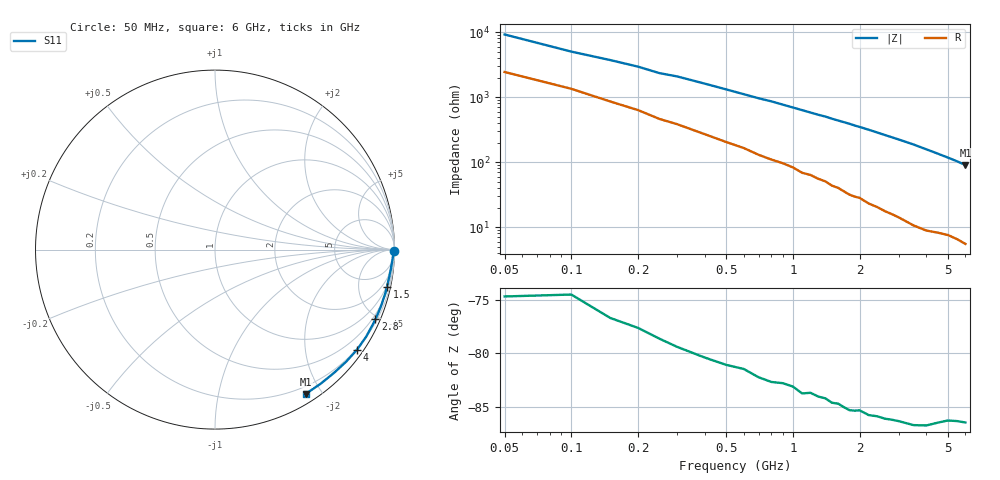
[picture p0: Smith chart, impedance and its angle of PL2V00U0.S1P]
! Infineon Technologies  Discrete & RF Semiconductors
! BAR 64-04W /-05W /-06W
! Si PIN Diode in SOT323
! VR = 2 V
! S-Parameters:  October  2008
# GHz  S  MA  R  50
!  f  S11
! GHz  MAG  ANG
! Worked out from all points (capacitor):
!   34 points, 50 MHz to 6 GHz, reference 50 ohm
!   read as one part to ground: C = 329 fF near 50 MHz
!   lowest |Z| = 90.3 ohm at 6 GHz (marker M1)
!   S11 on the Smith chart (normalised r, x): 50 MHz: open; 1.5 GHz: 0.87, -9.28; 2.8 GHz: 0.32, -4.81; 4 GHz: 0.18, -3.14; 6 GHz: 0.11, -1.80
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0.05  0.9971 -0.6
0.1  0.9947 -1.1
0.2  0.9927 -1.9
0.25  0.9916 -2.4
0.3  0.9912 -2.7
0.7  0.9861 -5.9
0.8  0.9854 -6.6
1  0.9829 -8.2
1.1  0.983 -9.0
1.2  0.9814 -9.8
1.3  0.981 -10.6
1.4  0.9804 -11.3
1.5  0.9804 -12.2
1.6  0.9795 -13.0
1.8  0.9797 -14.6
1.9  0.9786 -15.5
2  0.9775 -16.3
2.2  0.9776 -18.0
2.4  0.9761 -19.8
2.6  0.9755 -21.6
2.8  0.9742 -23.4
3  0.9733 -25.2
3.5  0.972 -29.9
4  0.968 -35.2
4.5  0.9612 -40.5
5  0.9547 -46.0
5.5  0.9514 -51.7
6  0.9495 -57.9
